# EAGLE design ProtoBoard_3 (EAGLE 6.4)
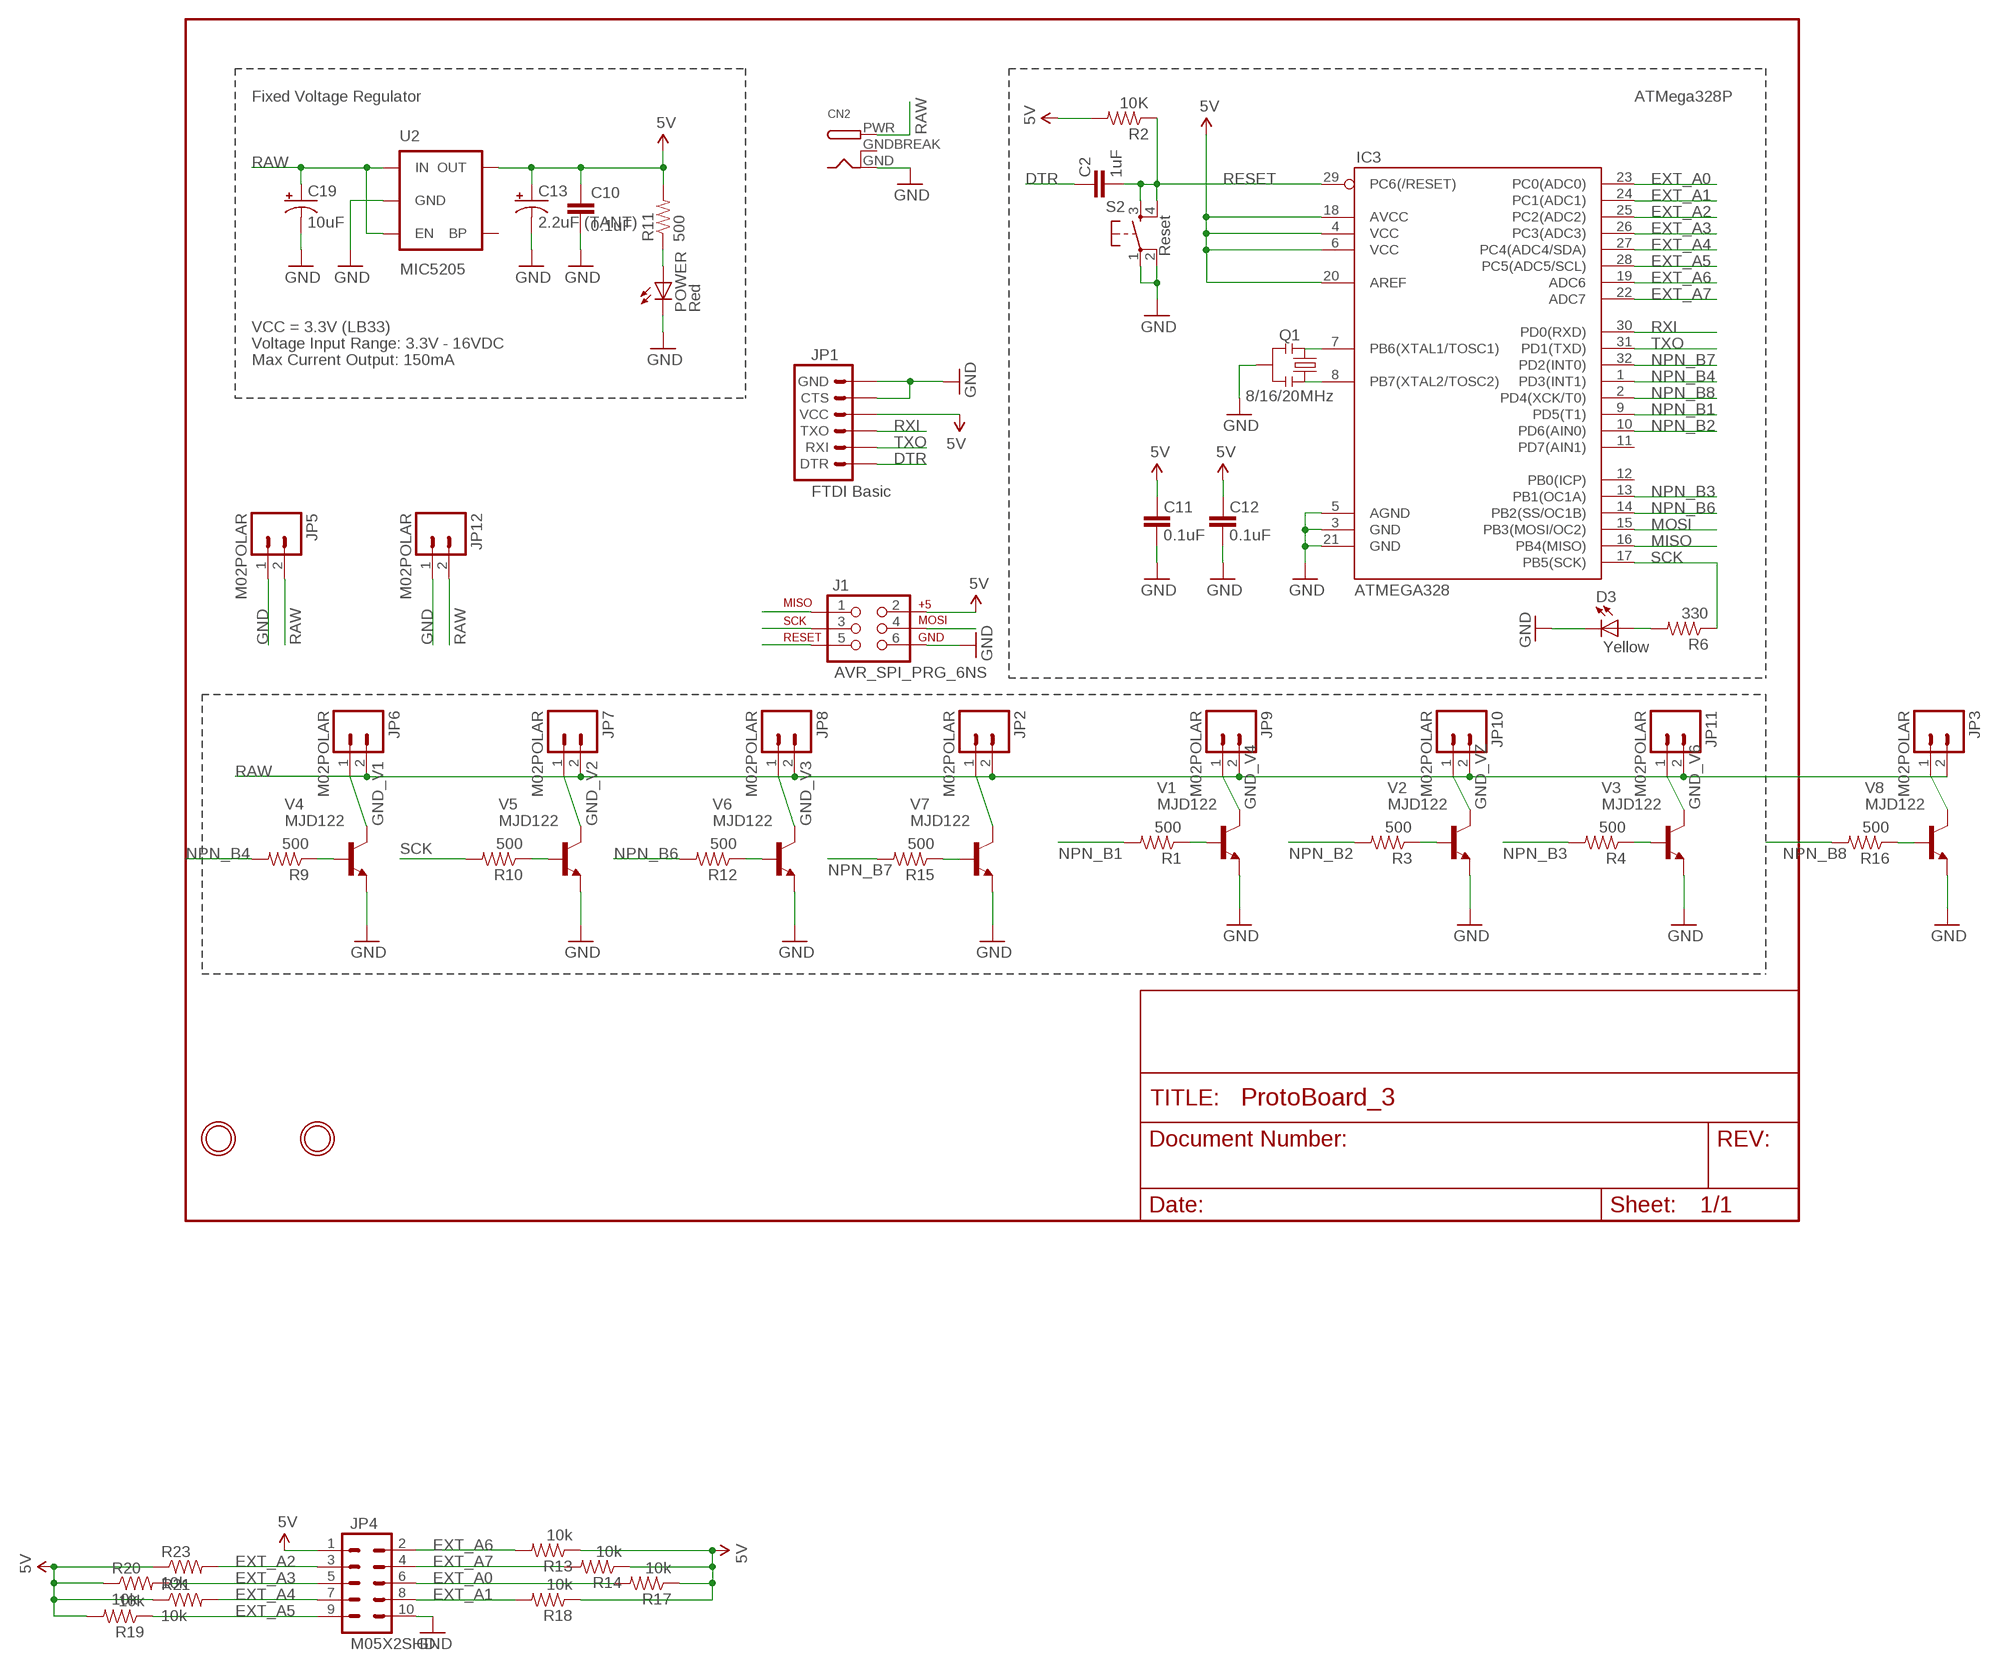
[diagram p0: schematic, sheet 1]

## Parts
C2  1uF  CAP0805  [0805]
C10  0.1uF  CAP0805  [0805]
C11  0.1uF  CAP0805  [0805]
C12  0.1uF  CAP0805  [0805]
C13  2.2uF (TANT)  CAP_POL1206  [EIA3216]
C19  10uF  CAP_POL1206  [EIA3216]
CN2  DCBARRELPTH  [DCJACK_2MM_PTH]
D3  Yellow  LED-YELLOWLILYPAD  [LED-1206]
IC3  ATMEGA328  ATMEGA168  [TQFP32-08]
J1  AVR_SPI_PRG_6NS  [2X3-NS]
JP1  FTDI Basic  ARDUINO_SERIAL_PROGRAMPTH  [1X06]
JP2  M02POLAR  [MOLEX-1X2]
JP3  M02POLAR  [MOLEX-1X2]
JP4  M05X2SHD  [2X5-SHROUDED]
JP5  M02POLAR  [MOLEX-1X2]
JP6  M02POLAR  [MOLEX-1X2]
JP7  M02POLAR  [MOLEX-1X2]
JP8  M02POLAR  [MOLEX-1X2]
JP9  M02POLAR  [MOLEX-1X2]
JP10  M02POLAR  [MOLEX-1X2]
JP11  M02POLAR  [MOLEX-1X2]
JP12  M02POLAR  [MOLEX-1X2]
POWER  Red  LED-RED1206  [LED-1206]
Q1  8/16/20MHz  RESONATORSMD  [RESONATOR-SMD]
R1  500  RESISTOR0805-RES  [0805]
R2  10K  RESISTOR0805-RES  [0805]
R3  500  RESISTOR0805-RES  [0805]
R4  500  RESISTOR0805-RES  [0805]
R6  330  RESISTOR0805-RES  [0805]
R9  500  RESISTOR0805-RES  [0805]
R10  500  RESISTOR0805-RES  [0805]
R11  500  RESISTOR0805-RES  [0805]
R12  500  RESISTOR0805-RES  [0805]
R13  10k  RESISTOR0805-RES  [0805]
R14  10k  RESISTOR0805-RES  [0805]
R15  500  RESISTOR0805-RES  [0805]
R16  500  RESISTOR0805-RES  [0805]
R17  10k  RESISTOR0805-RES  [0805]
R18  10k  RESISTOR0805-RES  [0805]
R19  10k  RESISTOR0805-RES  [0805]
R20  10k  RESISTOR0805-RES  [0805]
R21  10k  RESISTOR0805-RES  [0805]
R23  10k  RESISTOR0805-RES  [0805]
S2  Reset  TAC_SWITCHSMD  [TACTILE_SWITCH_SMD]
U2  MIC5205  V_REG_LDOSMD  [SOT23-5]
U$1  MOUNTINGHOLE2.5  [MOUNTINGHOLE_2.5_PLATED]
U$2  MOUNTINGHOLE2.5  [MOUNTINGHOLE_2.5_PLATED]
V1  MJD122  [DPAK]
V2  MJD122  [DPAK]
V3  MJD122  [DPAK]
V4  MJD122  [DPAK]
V5  MJD122  [DPAK]
V6  MJD122  [DPAK]
V7  MJD122  [DPAK]
V8  MJD122  [DPAK]

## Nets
5V: C10.1 C11.2 C12.2 C13.A(+) IC3.4(VCC) IC3.6(VCC) IC3.18(AVCC) IC3.20(AREF) J1.2 JP1.4(VCC) JP4.1 R2.2 R11.2 R13.1 R14.1 R17.1 R18.1 R19.2 R20.1 R21.1 R23.1 U2.5(OUT)
DTR: C2.2 JP1.1(DTR)
EXT_A0: IC3.23(PC0(ADC0)) JP4.6 R17.2
EXT_A1: IC3.24(PC1(ADC1)) JP4.8 R18.2
EXT_A2: IC3.25(PC2(ADC2)) JP4.3 R23.2
EXT_A3: IC3.26(PC3(ADC3)) JP4.5 R20.2
EXT_A4: IC3.27(PC4(ADC4/SDA)) JP4.7 R21.2
EXT_A5: IC3.28(PC5(ADC5/SCL)) JP4.9 R19.1
EXT_A6: IC3.19(ADC6) JP4.2 R13.2
EXT_A7: IC3.22(ADC7) JP4.4 R14.2
GND [vcc]: C10.2 C11.1 C12.1 C13.C(-) C19.C(-) CN2.GND D3.C IC3.3(GND) IC3.5(AGND) IC3.21(GND) J1.6 JP1.5(CTS) JP1.6(GND) JP4.10 JP5.1 JP12.1 POWER.C Q1.2 S2.1 S2.2 U2.2(GND) V1.3(E) V2.3(E) V3.3(E) V4.3(E) V5.3(E) V6.3(E) V7.3(E) V8.3(E)
GND_V1 [vcc]: JP6.1 V4.4(C)
GND_V2 [vcc]: JP7.1 V5.4(C)
GND_V3 [vcc]: JP8.1 V6.4(C)
GND_V4 [vcc]: JP9.1 V1.4(C)
GND_V6 [vcc]: JP11.1 V3.4(C)
GND_V7: JP2.1 V7.4(C)
GND_V8: JP3.1 V8.4(C)
GND_VZ [vcc]: JP10.1 V2.4(C)
MISO: IC3.16(PB4(MISO)) J1.1
MOSI: IC3.15(PB3(MOSI/OC2)) J1.4
N$1: IC3.8(PB7(XTAL2/TOSC2)) Q1.1
N$2: IC3.7(PB6(XTAL1/TOSC1)) Q1.3
N$3: R9.1 V4.1(B)
N$4: R1.1 V1.1(B)
N$5: R10.1 V5.1(B)
N$6: R12.1 V6.1(B)
N$7: D3.A R6.2
N$8: R3.1 V2.1(B)
N$11: R4.1 V3.1(B)
N$12: R16.1 V8.1(B)
N$14: R15.1 V7.1(B)
N$38: POWER.A R11.1
NPN_B1: IC3.9(PD5(T1)) R1.2
NPN_B2: IC3.10(PD6(AIN0)) R3.2
NPN_B3: IC3.13(PB1(OC1A)) R4.2
NPN_B4: IC3.1(PD3(INT1)) R9.2
NPN_B6: IC3.14(PB2(SS/OC1B)) R12.2
NPN_B7: IC3.32(PD2(INT0)) R15.2
NPN_B8: IC3.2(PD4(XCK/T0)) R16.2
RAW [vcc]: C19.A(+) CN2.PWR JP2.2 JP3.2 JP5.2 JP6.2 JP7.2 JP8.2 JP9.2 JP10.2 JP11.2 JP12.2 U2.1(IN) U2.3(EN)
RESET: C2.1 IC3.29(PC6(/RESET)) J1.5 R2.1 S2.3 S2.4
RXI: IC3.30(PD0(RXD)) JP1.3(TXO)
SCK: IC3.17(PB5(SCK)) J1.3 R6.1 R10.2
TXO: IC3.31(PD1(TXD)) JP1.2(RXI)
Unconnected: IC3.11(PD7(AIN1)) IC3.12(PB0(ICP)) U2.4(BP)

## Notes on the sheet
- Fixed Voltage Regulator | ATMega328P
- VCC = 3.3V (LB33)
- Voltage Input Range: 3.3V - 16VDC
- Max Current Output: 150mA

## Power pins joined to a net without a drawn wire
GNDBREAK: CN2.GNDBREAK

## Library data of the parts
C2 C10-C12 = SparkFun-Capacitors:CAP: Capacitor
C13 C19 = SparkFun:CAP_POL: Capacitor Polarized
CN2 = adafruit:DCBARREL: 2.0mm DC Barrel Jack DCJACK_2MM_PTH - Through Hole Jack (4UConnector: 05537)
D3 = SparkFun-LED:LED-YELLOW: Yellow SMD LEDs; PROD_ID: DIO-09909
IC3 = SparkFun:ATMEGA168
J1 = SparkFun-Connectors:AVR_SPI_PRG_6: AVR ISP 6 Pin This is the reduced ISP connector for AVR programming. Common on Arduino. This footprint will take up less PCB space and can be used with a 10-pin to 6-pin adapter such as SKU: BOB-08508
JP1 = SparkFun:ARDUINO_SERIAL_PROGRAM
JP2 JP3 JP5-JP12 = SparkFun-Connectors:M02: Standard 2-pin 0.1" header. Use with
JP4 = SparkFun-Connectors:M05X2: Header 5x2 Standard 10-pin dual row 0.1" header. Commonly used with AVR-ISP. Use with Spark Fun Electronics SKU: PRT-00778
POWER = SparkFun-LED:LED-RED: Assorted Red LEDs; PROD_ID: DIO-00809; VALUE: RED
Q1 = SparkFun:RESONATOR: Resonator Small SMD resonator. This is the itty bitty 10/20MHz resonators with built in caps. CSTCE10M0G55 and CSTCE20M0V53. Footprint has been reviewed closely but hasn't been tested yet.
R1-R4 R6 R9-R21 R23 = SparkFun-Resistors:RESISTOR: Resistor
S2 = SparkFun:TAC_SWITCH: Momentary Switch Button commonly used for reset or general input. Spark Fun Electronics SKU : COM-00097
U2 = SparkFun:V_REG_LDO: Voltage Regulator LDO Standard 150mA LDO voltage regulator in SOT-23 layout. Micrel part MIC5205. BP (by-pass) pin is used to lower output noise with 470pF cap.
U$1 U$2 = microbuilder:MOUNTINGHOLE: Mounting Hole
V1-V8 = digikey:MJD122

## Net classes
0 default: width 0.203 mm
1 vcc: width 0.254 mm

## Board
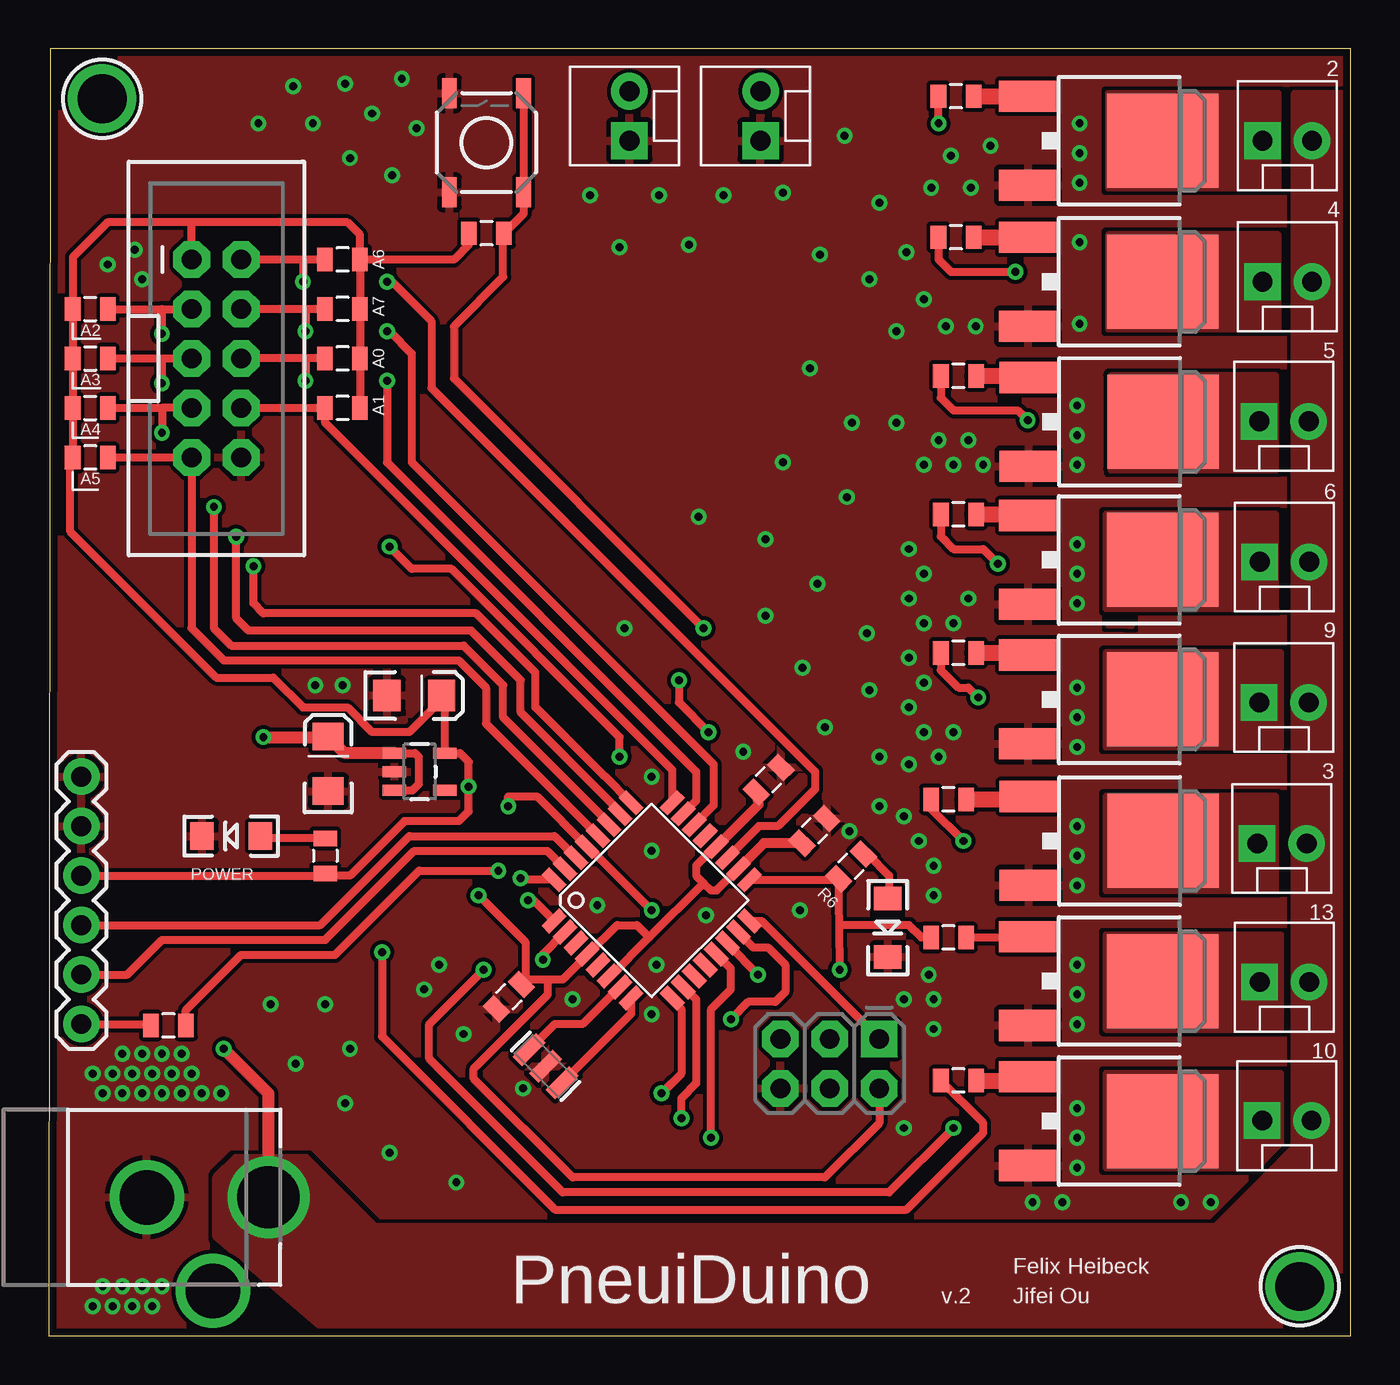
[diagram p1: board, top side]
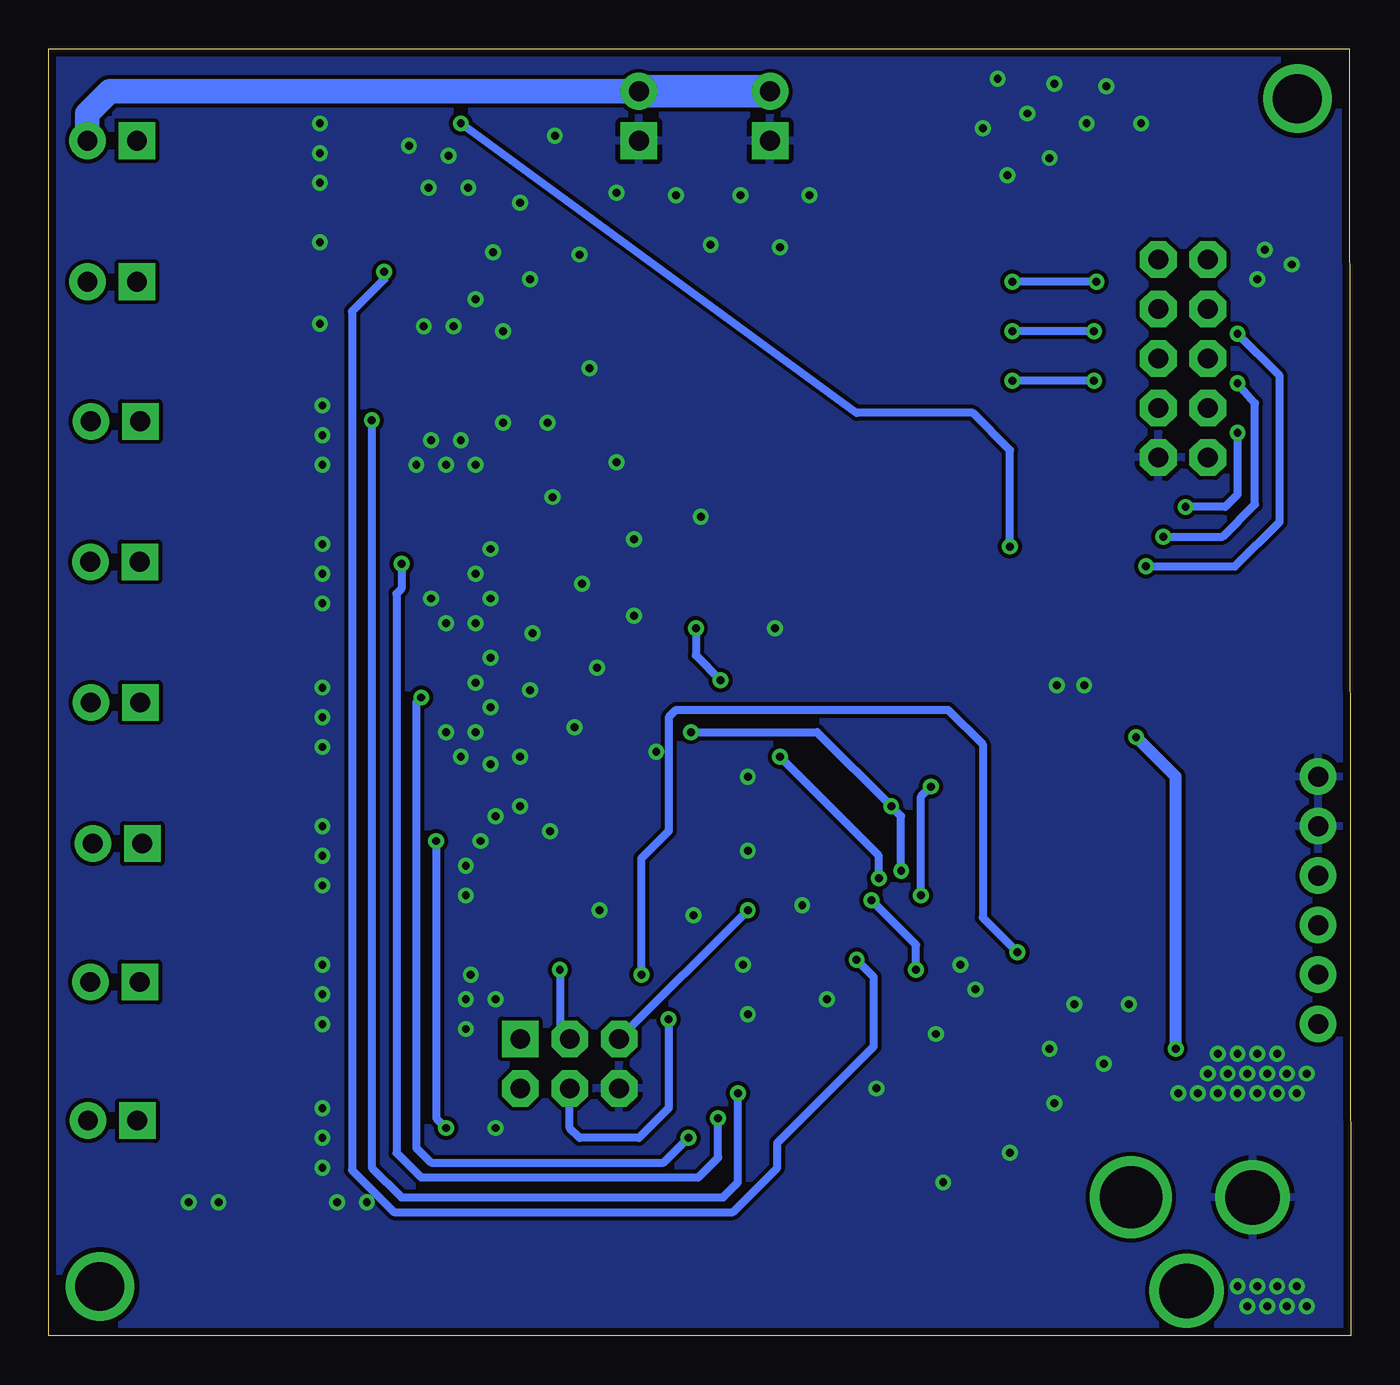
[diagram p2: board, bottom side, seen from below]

Size 66.86 x 66.07 mm. Coordinates in mm from the lower left corner, seen from the top.
Outline: 0,0 66.86,0 66.86,66.07 0.08,66.07 0,0
Copper layers (1*16): Top 0.035mm / dielectric 1.5mm / Bottom 0.035mm
Design rules "default *": minimum track width 10mil, minimum drill 16mil, track to track 8mil, track to pad 8mil, pad to pad 8mil, via to via 8mil, smd to smd 8mil, copper to edge 15mil, drill to drill 8mil, minimum pad ring 10mil, minimum via ring 8mil, stop-mask expansion 4mil, vias tented up to drill 17mil, thermal gap 10mil

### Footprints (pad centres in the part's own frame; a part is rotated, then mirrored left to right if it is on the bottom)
0805 = smd 0.8 x 1.2: 1 -0.9,0; 2 0.9,0
EIA3216 = smd 1.4 x 1.6: A 1.4,0; C -1.4,0
DCJACK_2MM_PTH = drill 2.8: GND 0,7.35; GNDBREAK 4.8,10.75 | drill 3.2: PWR 0,13.6
LED-1206 = smd 1.2 x 1.4: A -1.5,0; C 1.5,0
TQFP32-08 = smd 1.27 x 0.559: 1 -4.293,2.8; 2 -4.293,2; 3 -4.293,1.2; 4 -4.293,0.4; 5 -4.293,-0.4; 6 -4.293,-1.2; 7 -4.293,-2; 8 -4.293,-2.8; 17 4.293,-2.8; 18 4.293,-2; 19 4.293,-1.2; 20 4.293,-0.4; 21 4.293,0.4; 22 4.293,1.2; 23 4.293,2; 24 4.293,2.8 | smd 0.559 x 1.27: 9 -2.8,-4.293; 10 -2,-4.293; 11 -1.2,-4.293; 12 -0.4,-4.293; 13 0.4,-4.293; 14 1.2,-4.293; 15 2,-4.293; 16 2.8,-4.293; 25 2.8,4.293; 26 2,4.293; 27 1.2,4.293; 28 0.4,4.293; 29 -0.4,4.293; 30 -1.2,4.293; 31 -2,4.293; 32 -2.8,4.293
2X3-NS = drill 1.016 pad 1.88 square: 1 -2.54,-1.27 | drill 1.016 pad 1.88 octagon: 2 -2.54,1.27; 3 0,-1.27; 4 0,1.27; 5 2.54,-1.27; 6 2.54,1.27
1X06 = drill 1.016 pad 1.88: 1 0,0; 2 2.54,0; 3 5.08,0; 4 7.62,0; 5 10.16,0; 6 12.7,0
MOLEX-1X2 = drill 1.016 pad 1.88 square: 1 0,0 | drill 1.016 pad 1.88: 2 2.54,0
2X5-SHROUDED = drill 1.016 pad 1.88 octagon: 1 -1.27,5.08; 2 1.27,5.08; 3 -1.27,2.54; 4 1.27,2.54; 5 -1.27,0; 6 1.27,0; 7 -1.27,-2.54; 8 1.27,-2.54; 9 -1.27,-5.08; 10 1.27,-5.08
RESONATOR-SMD = smd 0.7 x 1.7: 1 -1.2,0; 2 0,0; 3 1.2,0
TACTILE_SWITCH_SMD = smd 1.524 x 0.762: 1 -2.54,1.905; 2 2.54,1.905; 3 -2.54,-1.905; 4 2.54,-1.905
SOT23-5 = smd 0.55 x 1.2: 1 -0.95,-1.3; 2 0,-1.3; 3 0.95,-1.3; 4 0.95,1.3; 5 -0.95,1.3
MOUNTINGHOLE_2.5_PLATED = drill 2.5 pad 3.2: P$1 0,0
DPAK = smd 1.6 x 3: 1 -2.28,-5.31; 3 2.28,-5.31 | smd 4.826 x 5.715: 4 0,1.588

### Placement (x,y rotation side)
C2  6.14,15.93 180 top
C10  23.63,17.41 225 top
C11  39.31,25.92 225 top
C12  36.96,28.54 225 top
C13  18.77,32.87 0 top
C19  14.35,29.36 90 top
CN2  -2.31,7.11 270 top
D3  43.08,20.95 270 top
IC3  30.96,22.35 45 top
J1  40.11,13.97 180 top
JP1  1.68,16 90 top
JP2  62.33,61.34 0 top
JP3  62.33,54.1 0 top
JP4  8.61,50.16 0 top
JP5  36.55,61.34 90 top
JP6  62.05,25.27 0 top
JP7  62.18,18.16 0 top
JP8  62.31,11.05 0 top
JP9  62.15,46.94 0 top
JP10  62.18,39.73 0 top
JP11  62.15,32.51 0 top
JP12  29.82,61.34 90 top
POWER  9.37,25.65 180 top
Q1  25.51,13.83 135 top
R1  46.71,49.28 180 top
R2  22.48,56.59 180 top
R3  46.71,42.16 180 top
R4  46.71,35.05 180 top
R6  41.2,24.1 45 top
R9  46.2,27.53 180 top
R10  46.2,20.45 180 top
R11  14.2,24.64 270 top
R12  46.71,13.11 180 top
R13  15.09,55.24 180 top
R14  15.09,52.7 180 top
R15  46.58,63.63 180 top
R16  46.58,56.39 180 top
R17  15.09,50.16 180 top
R18  15.09,47.62 180 top
R19  2.13,45.09 180 top
R20  2.13,50.16 0 top
R21  2.13,47.62 0 top
R23  2.13,52.7 0 top
S2  22.48,61.24 90 top
U2  19.05,28.96 270 top
U$1  2.74,63.5 0 top
U$2  64.24,2.54 0 top
V1  55.63,46.91 270 top
V2  55.6,39.83 270 top
V3  55.6,32.66 270 top
V4  55.63,25.4 270 top
V5  55.6,18.21 270 top
V6  55.6,11.02 270 top
V7  55.6,61.34 270 top
V8  55.6,54.1 270 top

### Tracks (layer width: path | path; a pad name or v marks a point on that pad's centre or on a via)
5V  (via drill 0.41)
  Top 0.406: IC3.20 34.22,25.1 33.25,24.13 33.25,23.62 33.63,23.24 | 33.63,23.24 34.01,22.86 34.3,22.86 IC3.18 | IC3.6 28.86,18.47 30.84,20.45 | 30.84,20.45 33.63,23.24 | 30.84,20.45 30.2,21.08 29.18,21.08 27.7,19.6 IC3.4 27.64,19.54 26.39,18.29 25.63,18.29 | 25.63,18.29 24.51,18.29 | 24.51,18.29 C10.1 | JP1.4 14.08,23.62 R11.2 14.31,23.62 15.47,23.62 18.26,26.42 21.06,26.42 21.56,26.92 v21.56,28.19 21.56,29.46 21.12,29.91 U2.5 20.35,32.69 C13.A 20.17,32.64 18.52,30.99 16.61,30.99 15.34,32.26 13.06,32.26 11.53,33.78 8.61,33.78 1.12,41.27 1.12,44.97 R19.2 R21.1 R20.1 R23.1 1.24,52.72 1.24,55.37 3.02,57.15 7.34,57.15 | 24.51,18.29 24.51,20.17 v22.07,22.61 | J1.2 42.65,10.92 39.85,8.13 26.9,8.13 21.82,13.21 21.82,13.72 25.63,17.53 25.63,18.29 | R13.1 R14.1 R17.1 R18.1 | R13.1 15.99,56.5 15.34,57.15 7.34,57.15 | R2.2 21.58,56.02 20.8,55.24 R13.1 | JP4.1 7.34,57.15
  Top 0.508: C12.2 36.45,27.27 IC3.20 | C11.2 36.72,25.28 IC3.18
  Bottom 0.406: v22.07,22.61 22.07,27.69 v21.56,28.19
DTR
  Top 0.406: JP1.1 5.17,16 C2.2
EXT_A0  (via drill 0.41)
  Top 0.406: 13.18,50.16 JP4.6 | R17.2 13.18,50.16 | 13.18,50.16 v13.18,49.02 | v17.37,49.02 17.37,44.83 33.25,28.96 33.25,27.47 IC3.23
  Bottom 0.406: v13.18,49.02 v17.37,49.02
EXT_A1
  Top 0.406: JP4.8 R18.2 14.2,47.61 14.2,46.86 32.02,29.04 IC3.24
EXT_A2  (via drill 0.41)
  Top 0.406: IC3.25 28.54,28.74 28.51,28.74 24.99,32.26 24.99,34.04 21.95,37.08 11.02,37.08 10.52,37.59 v10.52,39.5 | R23.2 5.82,52.7 | 5.82,52.7 JP4.3 | v5.82,51.44 5.82,52.7
  Bottom 0.406: v10.52,39.5 5.94,39.5 3.66,41.78 3.66,49.28 v5.82,51.44
EXT_A3  (via drill 0.41)
  Top 0.406: R20.2 5.94,50.16 | 5.94,50.16 JP4.5 | IC3.26 29.34,26.89 24.23,32 24.23,33.66 21.69,36.2 10.26,36.2 9.63,36.83 v9.63,41.02 | v5.82,48.9 5.82,50.04 5.94,50.16
  Bottom 0.406: v9.63,41.02 6.58,41.02 4.93,42.67 4.93,47.88 v5.82,48.9
EXT_A4  (via drill 0.41)
  Top 0.406: R21.2 5.82,47.62 | JP4.7 5.82,47.62 | 5.82,47.62 v5.82,46.35 | v8.48,42.55 8.48,36.32 9.37,35.43 21.31,35.43 23.34,33.4 23.34,31.75 28.78,26.32 IC3.27
  Bottom 0.406: v5.82,46.35 5.82,43.18 6.45,42.55 v8.48,42.55
EXT_A5
  Top 0.406: R19.1 JP4.9 7.34,36.32 8.99,34.67 21.06,34.67 22.45,33.27 22.45,31.43 IC3.28
EXT_A6  (via drill 0.41)
  Top 0.406: 13.06,55.24 JP4.2 | R13.2 13.06,55.24 | 13.06,55.24 v13.06,54.1 | v17.37,54.1 17.63,54.1 19.66,52.07 19.66,48.64 39.34,28.96 39.34,28.07 37.44,26.16 36.47,26.16 IC3.19
  Bottom 0.406: v13.06,54.1 v17.37,54.1
EXT_A7  (via drill 0.41)
  Top 0.406: 13.18,52.7 JP4.4 | R14.2 13.18,52.7 | 13.18,52.7 v13.18,51.56 | v17.37,51.56 17.5,51.56 18.64,50.42 18.64,44.83 34.14,29.34 34.14,27.22 IC3.22
  Bottom 0.406: v13.18,51.56 v17.37,51.56
GND  (via drill 0.41)
  other vias: 20.93,7.87 15.21,11.94 17.5,9.4 26.9,17.27 30.96,28.7 30.96,24.89 28.17,22.1 33.76,21.59 31.22,19.05 30.96,16.51 38.58,21.84 35.66,29.97 41.12,25.91 43.92,17.27 14.2,17.02 11.4,17.02 20.04,19.05 19.28,17.78 24.36,12.7 2.26,13.46 3.28,13.46 4.29,13.46 5.31,13.46 6.32,13.46 7.34,13.46 2.77,12.45 3.78,12.45 4.8,12.45 5.82,12.45 6.83,12.45 7.85,12.45 8.86,12.45 6.83,14.48 5.82,14.48 4.8,14.48 3.78,14.48 2.26,1.52 3.28,1.52 4.29,1.52 5.31,1.52 2.77,2.54 3.78,2.54 4.8,2.54 5.82,2.54 12.67,13.97 15.47,14.73 45.69,45.97 47.22,45.97 46.46,44.7 44.93,44.7 47.98,44.7 43.54,46.86 44.93,39.12 41.25,46.86 44.17,37.85 41,43.05 47.22,37.85 38.71,34.29 44.93,36.58 46.46,36.58 47.35,58.93 42.14,33.15 44.17,32.26 42.14,54.23 43.54,51.56 36.8,36.96 44.93,30.99 46.46,30.99 42.65,29.72 42.65,58.17 45.69,29.72 48.36,61.09 44.93,53.21 44.17,29.34 39.85,31.24 42.65,27.18 43.92,26.67 44.68,25.4 45.44,24.13 45.44,22.61 45.31,58.93 44.04,55.63 44.93,33.53 42.01,36.07 44.17,34.8 44.17,40.39 46.33,60.58 45.19,18.54 45.44,17.27 45.44,15.75 52.81,17.53 52.81,16 52.81,11.68 52.81,8.64 50.52,6.86 52.04,6.86 58.14,6.86 59.66,6.86 52.81,10.16 52.81,19.05 52.81,23.11 52.81,24.64 52.81,26.16 52.81,30.23 52.81,31.75 52.81,33.27 52.81,37.59 52.81,39.12 52.81,40.64 52.81,44.7 52.81,46.23 52.81,47.75 43.92,10.67 21.31,15.49 39.47,38.61 33.38,42.04 29.57,36.32 52.93,51.94 52.93,60.71 52.93,62.23 47.6,51.82 46.08,51.82 3.02,54.99 4.42,55.75 4.8,54.23 15.09,33.4 13.69,33.4 27.79,58.55 37.69,58.67 34.65,58.55 31.34,58.55 29.31,55.88 32.87,56.01 10.77,62.23 18.9,61.98 17.63,59.56 18.14,64.52 16.61,62.74 15.21,64.26 39.09,49.66 39.6,55.5 40.87,61.59 52.93,56.13 52.93,59.18 37.69,44.83 36.8,40.89 15.47,60.45 13.56,62.23 12.55,64.14
  pour Bottom (rank 3): -0.15,66.67 70.71,66.67 70.84,-0.76 -0.03,-0.76
  pour Top (rank 5): 0.61,67.44 70.97,67.44 70.33,-0.51 -0.03,-0.51
GND_V1
  pour Top (no thermals): 55.68,36.42 54.36,36.45 55.4,36.42
  pour Top (no thermals): 54.33,27.69 62.97,27.69 62.97,22.86 54.33,22.86
GND_V2
  pour Top (no thermals): 54.33,20.57 63.22,20.57 63.22,15.75 54.33,15.75
GND_V3
  pour Top (no thermals): 59.77,19.63 59.77,17.14 59.66,17.04 54.99,17.04 54.79,17.25 54.79,19.74
  pour Top (no thermals): 54.33,13.46 63.22,13.46 63.22,9.91 61.95,8.64 54.33,8.64
GND_V4
  pour Top (no thermals): 54.58,49.28 62.97,49.28 62.97,44.45 54.58,44.45
GND_V6
  pour Top (no thermals): 54.33,35.05 63.22,35.05 63.22,30.23 54.33,30.23
GND_V7
  pour Top (no thermals): 54.46,63.75 63.09,63.75 63.09,58.93 54.46,58.93
GND_V8
  pour Top (no thermals): 54.46,56.52 63.09,56.52 63.09,51.69 54.46,51.69
GND_VZ
  pour Top (no thermals): 54.33,42.16 62.97,42.16 62.97,37.34 54.33,37.34
MISO
  Top 0.406: IC3.16 36.59,21.3 J1.1
MOSI  (via drill 0.41)
  Top 0.406: IC3.15 35.41,20.7 36.17,19.94 36.93,19.94 37.82,19.05 37.82,17.65 37.31,17.14 35.92,17.14 v35.03,16.26
  Bottom 0.406: v35.03,16.26 35.03,11.68 36.55,10.16 39.6,10.16 40.11,10.67 J1.4
N$1
  Top 0.406: IC3.8 29.91,16.53 Q1.1
N$2
  Top 0.406: IC3.7 29.31,17.9 27.41,16 25.98,16 Q1.3
N$3
  Top 0.813: R9.1 50.17,27.53 V4.1
N$4
  Top 0.813: R1.1 50.23,49.28 V1.1
N$5
  Top 0.406: R10.1 50.25,20.45 V5.1
N$6
  Top 0.813: R12.1 50.09,13.11 V6.1
N$7
  Top 0.406: R6.2 42.04,24.74 43.15,23.62 43.15,22.52 D3.A
N$8
  Top 0.813: R3.1 50.23,42.16 V2.1
N$11
  Top 0.813: 50.52,35.05 50.77,34.8 50.44,34.8 V3.1 50.18,35.05 R4.1
N$12
  Top 0.813: R16.1 V8.1
N$14
  Top 0.813: R15.1 V7.1
N$38
  Top 0.406: R11.1 10.99,25.54 POWER.A
NPN_B1  (via drill 0.41)
  Top 0.406: R1.2 45.81,48.14 46.46,47.5 49.76,47.5 v50.27,46.99 | 32.02,12.99 v31.47,12.45 32.49,13.46 32.49,16.76 32.02,17.23 IC3.9
  Bottom 0.406: v50.27,46.99 50.27,8.64 48.74,7.11 32.23,7.11 31.47,7.87 v31.47,12.45
NPN_B2  (via drill 0.41)
  Top 0.406: R3.2 45.81,41.03 46.46,40.39 47.98,40.39 v48.74,39.62 | v32.49,11.18 32.49,12.19 33.25,12.95 33.25,17.27 32.62,17.9 IC3.10
  Bottom 0.406: v48.74,39.62 48.74,38.35 49,38.1 49,9.4 47.73,8.13 33.5,8.13 32.49,9.14 v32.49,11.18
NPN_B3  (via drill 0.41)
  Top 0.406: R4.2 45.81,34.17 46.71,33.27 47.22,33.27 v47.73,32.77 | v34.01,10.16 34.01,16.76 35.03,17.78 35.03,18.85 IC3.13
  Bottom 0.406: v47.73,32.77 47.98,32.51 47.98,9.65 47.22,8.89 35.28,8.89 v34.01,10.16
NPN_B4  (via drill 0.41)
  Top 0.406: R9.2 45.3,27.06 v46.96,25.4 | v46.46,10.67 43.15,7.37 26.39,7.37 19.53,14.22 19.53,16 v22.33,18.8 | v24.61,22.35 24.89,22.35 IC3.1
  Bottom 0.406: v46.96,25.4 46.96,11.18 v46.46,10.67 | v22.33,18.8 22.33,20.07 v24.61,22.35
NPN_B6  (via drill 0.41)
  Top 0.406: IC3.14 34.85,20.12 v36.42,18.54 | v17.12,19.68 17.12,15.37 26.01,6.48 44.04,6.48 47.98,10.41 47.98,10.94 R12.2
  Bottom 0.406: v36.42,18.54 36.42,24.51 35.03,25.91 35.03,31.75 34.65,32.13 20.68,32.13 18.9,30.35 18.9,21.46 v17.12,19.68
NPN_B7  (via drill 0.41)
  Top 0.406: IC3.32 24.32,23.41 v24.23,23.5 | v29.31,29.72 29.31,30.73 20.68,39.37 18.64,39.37 v17.5,40.51 | v45.69,62.23 R15.2
  Bottom 0.406: v24.23,23.5 24.23,24.64 v29.31,29.72 | v17.5,40.51 17.5,45.47 19.41,47.37 25.37,47.37 v45.69,62.23
NPN_B8  (via drill 0.41)
  Top 0.406: R16.2 45.68,55.26 46.33,54.61 v49.63,54.61 | v25.37,19.3 25.37,19.59 IC3.2
  Bottom 0.406: v25.37,19.3 24.49,18.41 24.49,14.86 29.44,9.91 29.44,8.64 31.72,6.35 49.12,6.35 51.28,8.51 51.28,52.58 49.63,54.23 v49.63,54.61
RAW  (via drill 0.41)
  Top 0.406: U2.1 18.81,29.91 19,29.72 19,28.32 18.67,27.99 17.77,27.99 U2.3
  Top 0.61: U2.1 15.21,29.91 C19.A 14.32,30.73 v11.02,30.73 | CN2.PWR 11.29,12.44 v8.99,14.73
  Bottom 0.61: v8.99,14.73 8.99,28.7 v11.02,30.73
  Bottom 1.27: JP5.2 63.73,63.88 64.87,62.74 JP2.2
  Bottom 1.676: JP12.2 JP5.2
  pour Top (no thermals): 16.74,5.59 59.92,5.59 63.98,9.65 63.98,63.75 68.55,63.75 68.81,0.51 13.94,0.51 8.61,5.08 8.61,8.13 9.63,9.14 13.18,9.14
RESET  (via drill 0.41)
  Top 0.406: v30.96,21.84 27.7,25.1 IC3.29 25.06,27.69 23.6,27.69 v23.6,27.18 | S2.4 S2.3 24.38,57.6 R2.1 23.34,56.55 23.34,54.36 20.8,51.82 20.8,49.15 v33.63,36.32 | C2.1 7.04,16.72 9.88,19.56 14.71,19.56 19.02,23.88 v23.09,23.88 | v32.36,33.66 32.36,32.51 v33.88,30.99
  Bottom 0.406: v30.96,21.84 J1.5 | v23.09,23.88 23.09,26.67 v23.6,27.18 27.41,30.99 v33.88,30.99 | v33.63,36.32 33.63,34.92 v32.36,33.66
RXI
  Top 0.406: JP1.3 13.94,21.08 18.52,25.65 25.96,25.65 IC3.30
SCK  (via drill 0.41)
  Top 0.406: IC3.17 40.51,23.41 R6.1 40.56,22.15 40.58,21.07 | 40.58,21.07 v40.61,18.8 | R10.2 44.81,20.45 44.17,21.08 40.59,21.08 40.58,21.07
  Bottom 0.406: v40.61,18.8 40.61,15.75 J1.3
TXO
  Top 0.406: JP1.2 4.04,18.54 5.82,20.32 14.2,20.32 18.77,24.89 25.59,24.89 IC3.31

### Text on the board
tNames: 2 | 4 | A6 | A7 | A2 | A0 | 5 | A3 | A1 | A4 | A5 | 6 | 9 | 3 | 13 | 10 | Felix Heibeck | PneuiDuino | v.2 | Jifei Ou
